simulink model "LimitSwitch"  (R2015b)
settings: Solver=VariableStepAuto  StartTime=0.0  StopTime=10.0  RelTol=1e-3
libraries: vexarmcortexlib x4

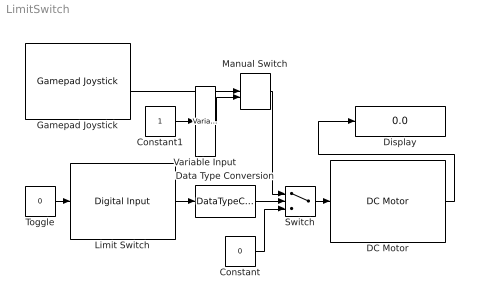
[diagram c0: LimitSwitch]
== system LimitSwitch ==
  Constant : Constant  Value=0
  Constant1 : Constant
  DC Motor : vexarmcortexlib/DC Motor  motor=5  scaleFactor=1/13.5  SimulationOut=on
  Data Type Conversion : DataTypeConversion  OutDataTypeStr=boolean
  Display : Display
  Gamepad Joystick : vexarmcortexlib/Gamepad Joystick  joystick=1  chan=2  SimulationIn=on
  Limit Switch : vexarmcortexlib/Digital Input  inChan=1  SimulationIn=on
  Manual Switch : ManualSwitch
  Switch : Switch
  Toggle : Constant  Value=0
  Variable Input : vexarmcortexlib/Utilities/Variable Input  low=-127  gain=127  high=127
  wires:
  DC Motor/1 -> Display/1
  Switch/1 -> DC Motor/1
  Constant/1 -> Switch/3
  Manual Switch/1 -> Switch/1
  Variable Input/1 -> Manual Switch/2
  Constant1/1 -> Variable Input/1
  Gamepad Joystick/1 -> Manual Switch/1
  Toggle/1 -> Limit Switch/1
  Limit Switch/1 -> Data Type Conversion/1
  Data Type Conversion/1 -> Switch/2
